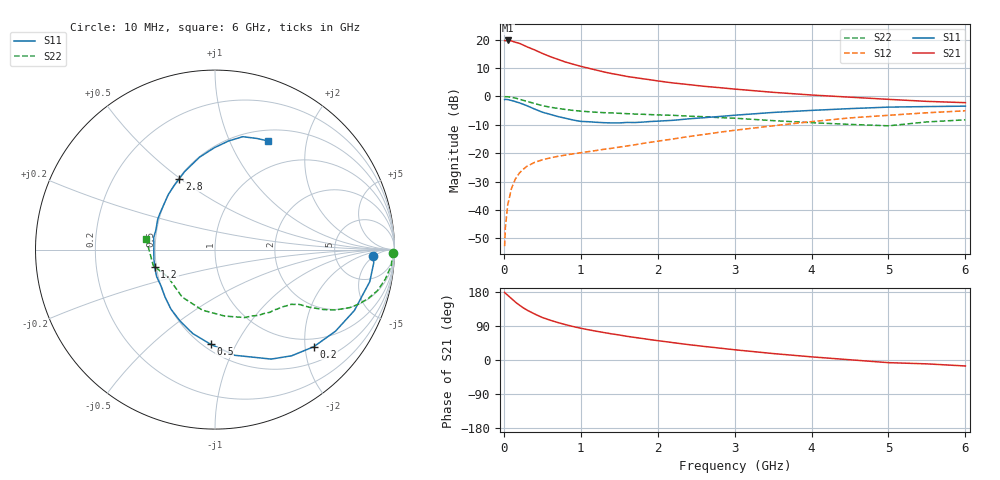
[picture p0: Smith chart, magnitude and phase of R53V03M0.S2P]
! SIEMENS Small Signal Semiconductors
! BFR183
! Si NPN RF Bipolar Junction Transistor in SOT23
! VCE = 3 V  IC = 3 mA
! Common Emitter S-Parameters:  May  1996
# GHz  S  MA  R  50
!  f  S11  S21  S12  S22
! GHz  MAG  ANG  MAG  ANG  MAG  ANG  MAG  ANG
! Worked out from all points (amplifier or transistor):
!   36 points, 10 MHz to 6 GHz, reference 50 ohm
!   highest |S21| = 19.7 dB at 50 MHz (marker M1)
!   |S21| within 3 dB of that: start of sweep to 370.5 MHz
!   unconditionally stable (mu >= 1): 1.238 GHz to 2.744 GHz
!   at 250 MHz: K = 0.30, MSG = 21.9 dB, |S12| = -25.7 dB
!   at 1.4 GHz: K = 1.05, MAG = 11.8 dB, |S12| = -18.3 dB
!   at 6 GHz: K = 0.89, MSG = 1.4 dB, |S12| = -5.1 dB
!   lowest NFmin = 1.10 dB at 450 MHz
!   S11 on the Smith chart (normalised r, x): 10 MHz: 14, -5; 200 MHz: 0.82, -2.19; 500 MHz: 0.54, -0.79; 1.2 GHz: 0.49, -0.11; 2.8 GHz: 0.51, +0.50; 6 GHz: 0.63, +1.41
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0.01  0.8798 -2.4  9.643 178.4  0.0023 87.2  0.9938 -1.0
0.02  0.8877 -4.7  9.568 176.2  0.0049 90.1  0.9871 -2.0
0.05  0.8806 -11.7  9.682 170.9  0.0122 84.7  0.987 -5.0
0.1  0.8475 -23.6  9.474 162.0  0.0241 76.9  0.9634 -9.8
0.15  0.8108 -34.1  8.998 152.9  0.035 71.6  0.9344 -14.1
0.2  0.7718 -44.5  8.637 145.1  0.0443 67.3  0.8962 -17.7
0.25  0.7295 -54.2  8.061 138.1  0.0519 62.5  0.8542 -20.9
0.3  0.6858 -62.8  7.491 131.8  0.0587 59.6  0.8191 -23.2
0.4  0.5988 -79.5  6.604 121.4  0.0688 54.7  0.7492 -26.7
0.5  0.5278 -92.7  5.726 112.2  0.0764 51.2  0.6885 -29.0
0.6  0.484 -104.8  5.047 105.2  0.0823 49.8  0.6467 -30.3
0.8  0.4126 -126.5  4.042 93.4  0.0925 48.1  0.5894 -32.2
0.9  0.3839 -136.4  3.694 88.3  0.0975 48.7  0.5669 -32.8
1.1  0.3582 -155.1  3.142 79.8  0.1066 50.0  0.5379 -34.6
1.2  0.3503 -163.7  2.914 76.0  0.1115 50.7  0.5264 -35.4
1.6  0.3482 168.9  2.249 62.5  0.1341 52.9  0.497 -39.7
2.2  0.3795 138.8  1.727 45.8  0.1781 55.2  0.4647 -48.7
2.8  0.4426 116.6  1.429 31.5  0.2336 53.5  0.4229 -60.9
3.5  0.522 99.5  1.181 17.0  0.3036 47.7  0.3743 -81.7
4.5  0.6098 82.9  0.97 0.6  0.4184 36.0  0.3216 -124.7
5.5  0.6622 69.2  0.818 -10.2  0.5152 22.6  0.3554 -165.6
6  0.6737 63.9  0.776 -15.8  0.5581 13.8  0.387 171.6
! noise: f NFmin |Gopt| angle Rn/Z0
0.45  1.1  0.37  35  0.3
0.9  1.15  0.34  85  0.23
1.8  1.9  0.35  160  0.13
